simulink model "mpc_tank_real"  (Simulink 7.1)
settings: Solver=ode45  StartTime=0.0  StopTime=300  RelTol=1e-3
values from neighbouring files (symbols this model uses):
  h1 = 10    [mpc_controller.m]
  h2 = 10    [mpc_controller.m]
  h3 = (k2*v2*(1-g2)/a3)^2/(2*g)    [mpc_controller.m]
  h4 = (k1*v1*(1-g1)/a4)^2/(2*g)    [mpc_controller.m]
  kc = 0.5    [mpc_controller.m]
  md = MPCInit(Ad,Bd,Cyd,Czd,Dzd,Ccd,Dcd,Hp,Hw,zblk,Hu,ublk,  	    du_max,du_min,u_max,u_min,z_max,  	    z_min,Q,R,W,V,Ts,2,'qp_as')    [mpc_controller.m]
  Tf1 = 0.5    [mpc_controller.m]
  Tf2 = 0.5    [mpc_controller.m]
  v1 = sqrt(2*g)*((g2-1)*a2*sqrt(h2)+g2*a1*sqrt(h1))/(k1*(g1+g2-1))    [mpc_controller.m]
  v2 = sqrt(2*g)*((g1-1)*a1*sqrt(h1)+g1*a2*sqrt(h2))/(k2*(g1+g2-1))    [mpc_controller.m]

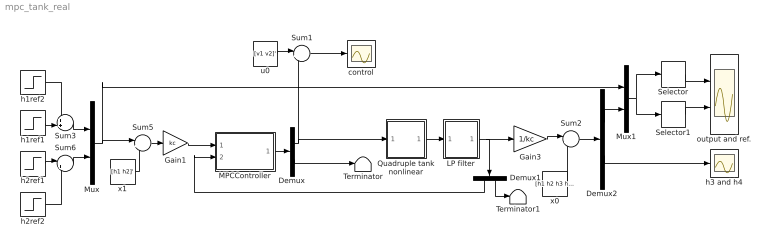
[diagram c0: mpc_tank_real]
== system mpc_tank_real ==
  Demux : Demux  Outputs=[md.m md.ne]
  Demux1 : Demux  Orientation=down  Outputs=[2 2]
  Demux2 : Demux  Outputs=[2 2]
  Gain1 : Gain  Gain=kc  ParameterDataType=sfix(16)  ParameterScaling=2^0  OutDataType=sfix(16)  OutScaling=2^0
  Gain3 : Gain  Gain=1/kc  ParameterDataType=sfix(16)  ParameterScaling=2^0  OutDataType=sfix(16)  OutScaling=2^0
  LP filter : Subsystem
  MPCController : Subsystem  mask{md=md}
      mask prompts: md "MPCData"
  Mux : Mux  Inputs=2
  Mux1 : Mux  Inputs=2
  Quadruple tank nonlinear : Subsystem
  Selector : Selector  InputPortWidth=4  IndexOptions=Index vector (dialog)  Indices=[1 3]  OutputSizes=1
  Selector1 : Selector  InputPortWidth=4  IndexOptions=Index vector (dialog)  Indices=[2 4]  OutputSizes=1
  Sum1 : Sum  Inputs=|++  OutDataType=sfix(16)  OutScaling=2^0
  Sum2 : Sum  Inputs=|++  OutDataType=sfix(16)  OutScaling=2^0
  Sum3 : Sum  Inputs=++|  OutDataType=sfix(16)  OutScaling=2^0
  Sum5 : Sum  Inputs=|+-  OutDataType=sfix(16)  OutScaling=2^0
  Sum6 : Sum  Inputs=|++  OutDataType=sfix(16)  OutScaling=2^0
  Terminator : Terminator
  Terminator1 : Terminator
  control : Scope
  h1ref1 : Step  Time=0  After=h1+1
  h1ref2 : Step  Time=120  After=3
  h2ref1 : Step  Time=0  After=h2+3
  h2ref2 : Step  Time=220
  h3 and h4 : Scope
  output and ref. : Scope  NumInputPorts=2
  u0 : Constant  Value=[v1 v2]'  OutDataType=sfix(16)  OutScaling=2^0
  x0 : Constant  Value=[h1 h2 h3 h4]'  OutDataType=sfix(16)  OutScaling=2^0
  x1 : Constant  Value=[h1 h2]'  OutDataType=sfix(16)  OutScaling=2^0
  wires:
  MPCController/1(u) -> Demux/1
  Demux/1 -> Sum1/2, Quadruple tank nonlinear/1(u)
  Demux/2 -> Terminator/1
  x1/1 -> Sum5/2
  Mux/1 -> Sum5/1, Mux1/1
  Sum5/1 -> Gain1/1
  u0/1 -> Sum1/1
  Sum1/1 -> control/1
  Gain3/1 -> Sum2/1
  x0/1 -> Sum2/2
  Quadruple tank nonlinear/1(y) -> LP filter/1(y)
  h1ref1/1 -> Sum3/2
  h2ref1/1 -> Sum6/1
  h2ref2/1 -> Sum6/2
  h1ref2/1 -> Sum3/1
  Demux1/2 -> Terminator1/1
  Sum2/1 -> Demux2/1
  Demux2/2 -> h3 and h4/1
  Demux2/1 -> Mux1/2
  Mux1/1 -> Selector/1, Selector1/1
  Selector/1 -> output and ref./1
  Selector1/1 -> output and ref./2
  Sum6/1 -> Mux/2
  Sum3/1 -> Mux/1
  Gain1/1 -> MPCController/1(Reference)
  Demux1/1 -> MPCController/2(Measurements)
  LP filter/1(yf) -> Gain3/1, Demux1/1

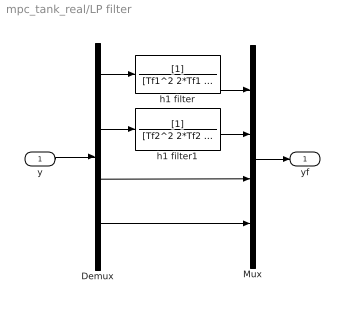
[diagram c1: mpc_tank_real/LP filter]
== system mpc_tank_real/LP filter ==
  y : Inport
  Demux : Demux
  Mux : Mux
  h1 filter : TransferFcn  Denominator=[Tf1^2 2*Tf1 1]
  h1 filter1 : TransferFcn  Denominator=[Tf2^2 2*Tf2 1]
  yf : Outport
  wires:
  Demux/4 -> Mux/4
  Demux/3 -> Mux/3
  Demux/1 -> h1 filter/1
  h1 filter/1 -> Mux/1
  Demux/2 -> h1 filter1/1
  h1 filter1/1 -> Mux/2
  Mux/1 -> yf/1
  y/1 -> Demux/1

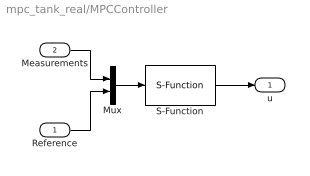
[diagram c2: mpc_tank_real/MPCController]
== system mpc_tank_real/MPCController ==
  Reference : Inport  OutDataType=sfix(16)  OutScaling=2^0
  Measurements : Inport  Port=2  OutDataType=sfix(16)  OutScaling=2^0
  Mux : Mux  Inputs=2
  S-Function : S-Function  FunctionName=MPCController  Parameters=md  EnableBusSupport=off
  u : Outport  OutDataType=sfix(16)  OutScaling=2^0
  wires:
  S-Function/1 -> u/1
  Reference/1 -> Mux/2
  Measurements/1 -> Mux/1
  Mux/1 -> S-Function/1

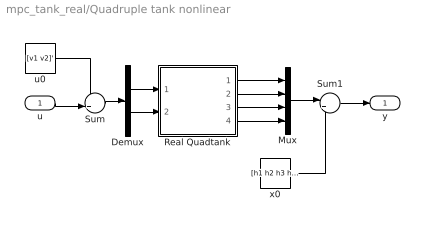
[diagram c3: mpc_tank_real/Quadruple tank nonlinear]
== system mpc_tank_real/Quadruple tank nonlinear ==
  u : Inport  OutDataType=sfix(16)  OutScaling=2^0
  Demux : Demux  Outputs=2
  Mux : Mux
  Real Quadtank : Subsystem  AncestorBlock=tank/Real Quadtank  mask{h=0.05}
  Sum : Sum  Inputs=++|  OutDataType=sfix(16)  OutScaling=2^0
  Sum1 : Sum  Inputs=|+-  OutDataType=sfix(16)  OutScaling=2^0
  u0 : Constant  Value=[v1 v2]'  OutDataType=sfix(16)  OutScaling=2^0
  x0 : Constant  Value=[h1 h2 h3 h4]*kc'  OutDataType=sfix(16)  OutScaling=2^0
  y : Outport  OutDataType=sfix(16)  OutScaling=2^0
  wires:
  Demux/1 -> Real Quadtank/1(u1)
  Demux/2 -> Real Quadtank/2(u2)
  Sum/1 -> Demux/1
  u0/1 -> Sum/1
  u/1 -> Sum/2
  x0/1 -> Sum1/2
  Sum1/1 -> y/1
  Mux/1 -> Sum1/1
  Real Quadtank/1(y1) -> Mux/1
  Real Quadtank/2(y2) -> Mux/2
  Real Quadtank/3(y3) -> Mux/3
  Real Quadtank/4(y4) -> Mux/4

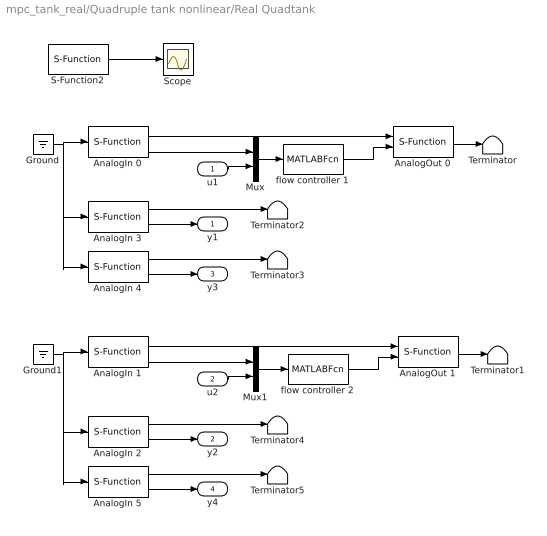
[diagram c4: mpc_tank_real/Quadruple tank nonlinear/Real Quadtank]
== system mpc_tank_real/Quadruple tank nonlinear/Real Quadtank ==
  u1 : Inport  OutDataType=sfix(16)  OutScaling=2^0
  u2 : Inport  Port=2  OutDataType=sfix(16)  OutScaling=2^0
  AnalogIn 0 : S-Function  FunctionName=analogin  Parameters=h [35]  EnableBusSupport=off
  AnalogIn 1 : S-Function  FunctionName=analogin  Parameters=h [34]  EnableBusSupport=off
  AnalogIn 2 : S-Function  FunctionName=analogin  Parameters=h [33]  EnableBusSupport=off
  AnalogIn 3 : S-Function  FunctionName=analogin  Parameters=h [31]  EnableBusSupport=off
  AnalogIn 4 : S-Function  FunctionName=analogin  Parameters=h [30]  EnableBusSupport=off
  AnalogIn 5 : S-Function  FunctionName=analogin  Parameters=h [32]  EnableBusSupport=off
  AnalogOut 0 : S-Function  FunctionName=analogout  Parameters=h [31]  EnableBusSupport=off
  AnalogOut 1 : S-Function  FunctionName=analogout  Parameters=h [30]  EnableBusSupport=off
  Ground : Ground
  Ground1 : Ground
  Mux : Mux  Inputs=2
  Mux1 : Mux  Inputs=2
  S-Function2 : S-Function  FunctionName=realtimer  Parameters=h  EnableBusSupport=off
  Scope : Scope
  Terminator{,1..5} (6 alike) : Terminator
  flow controller 1 : MATLABFcn  MATLABFcn=flowCtrl1  SampleTime=0.01
  flow controller 2 : MATLABFcn  MATLABFcn=flowCtrl2  SampleTime=0.01
  y1 : Outport  OutDataType=sfix(16)  OutScaling=2^0
  y2 : Outport  Port=2  OutDataType=sfix(16)  OutScaling=2^0
  y3 : Outport  Port=3  OutDataType=sfix(16)  OutScaling=2^0
  y4 : Outport  Port=4  OutDataType=sfix(16)  OutScaling=2^0
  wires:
  S-Function2/1 -> Scope/1
  AnalogIn 0/1 -> AnalogOut 0/1
  AnalogOut 0/1 -> Terminator/1
  AnalogIn 1/1 -> AnalogOut 1/1
  AnalogOut 1/1 -> Terminator1/1
  AnalogIn 3/2 -> y1/1
  AnalogIn 4/2 -> y3/1
  Ground/1 -> AnalogIn 0/1, AnalogIn 3/1, AnalogIn 4/1
  AnalogIn 3/1 -> Terminator2/1
  AnalogIn 4/1 -> Terminator3/1
  AnalogIn 2/2 -> y2/1
  AnalogIn 5/2 -> y4/1
  Ground1/1 -> AnalogIn 5/1, AnalogIn 2/1, AnalogIn 1/1
  AnalogIn 2/1 -> Terminator4/1
  AnalogIn 5/1 -> Terminator5/1
  u1/1 -> Mux/2
  Mux/1 -> flow controller 1/1
  flow controller 1/1 -> AnalogOut 0/2
  u2/1 -> Mux1/2
  Mux1/1 -> flow controller 2/1
  flow controller 2/1 -> AnalogOut 1/2
  AnalogIn 1/2 -> Mux1/1
  AnalogIn 0/2 -> Mux/1
